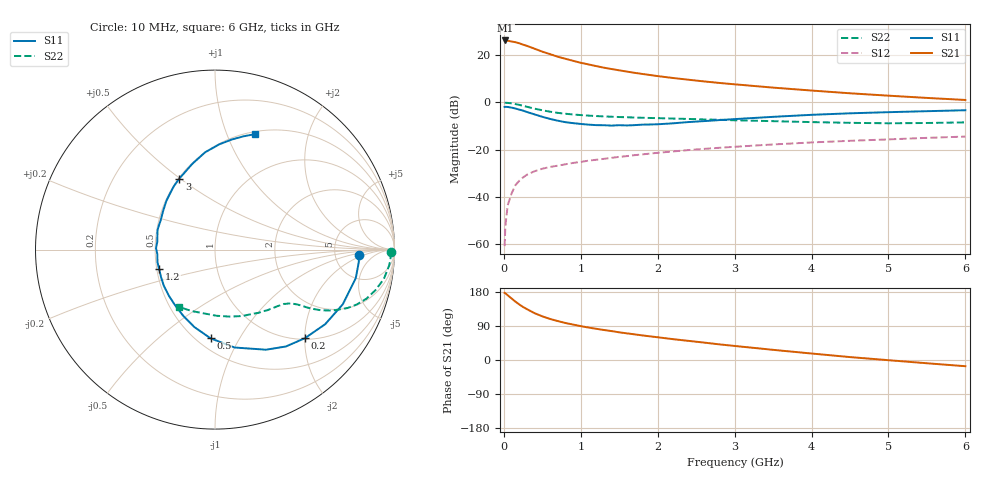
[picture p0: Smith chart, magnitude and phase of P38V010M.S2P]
! SIEMENS Small Signal Semiconductors
! BFP181
! Si NPN RF Bipolar Junction Transistor in SOT143
! VCE = 8 V  IC = 10 mA
! Common Emitter S-Parameters:  March  1996
# GHz  S  MA  R  50
!  f  S11  S21  S12  S22
! GHz  MAG  ANG  MAG  ANG  MAG  ANG  MAG  ANG
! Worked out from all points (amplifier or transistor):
!   36 points, 10 MHz to 6 GHz, reference 50 ohm
!   highest |S21| = 26.2 dB at 20 MHz (marker M1)
!   |S21| within 3 dB of that: start of sweep to 358.3 MHz
!   unconditionally stable (mu >= 1): 1.343 GHz to end of sweep
!   at 250 MHz: K = 0.30, MSG = 28.1 dB, |S12| = -31.8 dB
!   at 1.4 GHz: K = 1.01, MAG = 18.1 dB, |S12| = -23.5 dB
!   at 6 GHz: K = 1.03, MAG = 6.7 dB, |S12| = -14.5 dB
!   S11 on the Smith chart (normalised r, x): 10 MHz: 8.75, -1.57; 200 MHz: 1.03, -2.00; 500 MHz: 0.58, -0.76; 1.2 GHz: 0.51, -0.12; 3 GHz: 0.50, +0.50; 6 GHz: 0.53, +1.27
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0.01  0.8007 -2.3  20.49 177.2  0.0009 80.6  0.9808 -0.8
0.02  0.8042 -4.9  20.49 176.1  0.0024 84.2  0.981 -1.9
0.05  0.8003 -11.5  20.23 170.8  0.0066 87.6  0.9749 -5.1
0.1  0.7743 -23.2  19.49 162.5  0.0117 77.6  0.9547 -9.9
0.15  0.7413 -34.1  18.84 154.1  0.0176 72.2  0.922 -14.2
0.2  0.7032 -44.6  17.87 146.7  0.0218 68.4  0.8863 -18.0
0.25  0.6689 -53.8  16.71 139.9  0.0257 64.8  0.8466 -21.2
0.3  0.626 -63.0  15.74 134.2  0.0294 61.3  0.8068 -23.8
0.4  0.5563 -78.7  13.69 123.5  0.0348 56.7  0.7361 -27.5
0.5  0.4947 -92.9  11.87 115.2  0.0393 53.0  0.6801 -29.8
0.6  0.4467 -104.9  10.52 108.4  0.0429 51.5  0.6351 -31.3
0.7  0.4099 -115.4  9.272 102.8  0.0456 50.4  0.6005 -32.3
0.8  0.3808 -126.0  8.389 97.7  0.0488 49.3  0.5747 -32.9
1.1  0.3378 -152.8  6.372 85.6  0.0583 48.3  0.5244 -35.0
1.2  0.3297 -161.1  5.87 82.4  0.0609 48.1  0.5135 -35.8
1.7  0.3296 166.8  4.226 67.7  0.0762 47.1  0.4778 -40.4
2.2  0.3602 143.4  3.284 55.0  0.0914 44.6  0.4539 -46.5
3  0.4427 116.7  2.415 37.1  0.1146 39.4  0.4175 -58.6
3.5  0.4938 104.9  2.054 26.8  0.1285 35.9  0.4001 -67.7
4.5  0.5868 87.7  1.558 7.7  0.1534 27.9  0.3689 -88.5
5.5  0.6507 75.9  1.243 -8.6  0.1772 20.9  0.366 -110.7
6  0.6814 70.8  1.125 -16.4  0.1889 16.9  0.3773 -122.1
